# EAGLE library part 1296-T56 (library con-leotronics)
1.27mm SINGLE ROW FEMALE SOCKET Source: http://www.leotronics.co.uk/Conexcon/Data%20Sheets/sec.%20A/1296ing.pdf
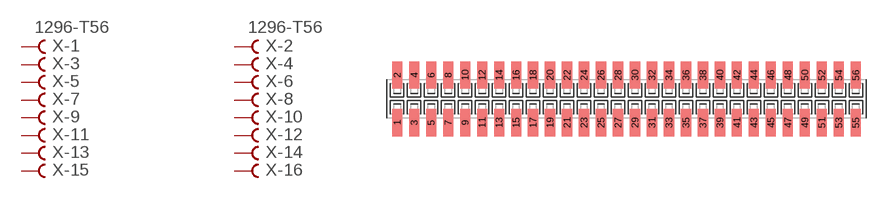
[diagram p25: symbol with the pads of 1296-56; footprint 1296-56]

Designator prefix X; gates -1=FVAL -2=FVAL -3=F -4=F -5=F -6=F -7=F -8=F -9=F -10=F -11=F -12=F -13=F -14=F -15=F -16=F -17=F -18=F -19=F -20=F -21=F -22=F -23=F -24=F -25=F -26=F -27=F -28=F -29=F -30=F -31=F -32=F -33=F -34=F -35=F -36=F -37=F -38=F -39=F -40=F -41=F -42=F -43=F -44=F -45=F -46=F -47=F -48=F -49=F -50=F -51=F -52=F -53=F -54=F -55=F -56=F

## 1296-T56 (OC_FARNELL: unknown; OC_NEWARK: unknown)  [1296-56]
1  -1:B  pas
2  -2:B  pas
3  -3:B  pas
4  -4:B  pas
5  -5:B  pas
6  -6:B  pas
7  -7:B  pas
8  -8:B  pas
9  -9:B  pas
10  -10:B  pas
11  -11:B  pas
12  -12:B  pas
13  -13:B  pas
14  -14:B  pas
15  -15:B  pas
16  -16:B  pas
17  -17:B  pas
18  -18:B  pas
19  -19:B  pas
20  -20:B  pas
21  -21:B  pas
22  -22:B  pas
23  -23:B  pas
24  -24:B  pas
25  -25:B  pas
26  -26:B  pas
27  -27:B  pas
28  -28:B  pas
29  -29:B  pas
30  -30:B  pas
31  -31:B  pas
32  -32:B  pas
33  -33:B  pas
34  -34:B  pas
35  -35:B  pas
36  -36:B  pas
37  -37:B  pas
38  -38:B  pas
39  -39:B  pas
40  -40:B  pas
41  -41:B  pas
42  -42:B  pas
43  -43:B  pas
44  -44:B  pas
45  -45:B  pas
46  -46:B  pas
47  -47:B  pas
48  -48:B  pas
49  -49:B  pas
50  -50:B  pas
51  -51:B  pas
52  -52:B  pas
53  -53:B  pas
54  -54:B  pas
55  -55:B  pas
56  -56:B  pas

## Footprint 1296-56 (pad centres in mm)
1.27mm SINGLE ROW FEMALE SOCKET Source: http://www.leotronics.co.uk/Conexcon/Data%20Sheets/sec.%20A/1296ing.pdf
smd 0.76 x 2.05: 1 -17.145,-1.78; 2 -17.145,1.78; 3 -15.875,-1.78; 4 -15.875,1.78; 5 -14.605,-1.78; 6 -14.605,1.78; 7 -13.335,-1.78; 8 -13.335,1.78; 9 -12.065,-1.78; 10 -12.065,1.78; 11 -10.795,-1.78; 12 -10.795,1.78; 13 -9.525,-1.78; 14 -9.525,1.78; 15 -8.255,-1.78; 16 -8.255,1.78; 17 -6.985,-1.78; 18 -6.985,1.78; 19 -5.715,-1.78; 20 -5.715,1.78; 21 -4.445,-1.78; 22 -4.445,1.78; 23 -3.175,-1.78; 24 -3.175,1.78; 25 -1.905,-1.78; 26 -1.905,1.78; 27 -0.635,-1.78; 28 -0.635,1.78; 29 0.635,-1.78; 30 0.635,1.78; 31 1.905,-1.78; 32 1.905,1.78; 33 3.175,-1.78; 34 3.175,1.78; 35 4.445,-1.78; 36 4.445,1.78; 37 5.715,-1.78; 38 5.715,1.78; 39 6.985,-1.78; 40 6.985,1.78; 41 8.255,-1.78; 42 8.255,1.78; 43 9.525,-1.78; 44 9.525,1.78; 45 10.795,-1.78; 46 10.795,1.78; 47 12.065,-1.78; 48 12.065,1.78; 49 13.335,-1.78; 50 13.335,1.78; 51 14.605,-1.78; 52 14.605,1.78; 53 15.875,-1.78; 54 15.875,1.78; 55 17.145,-1.78; 56 17.145,1.78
